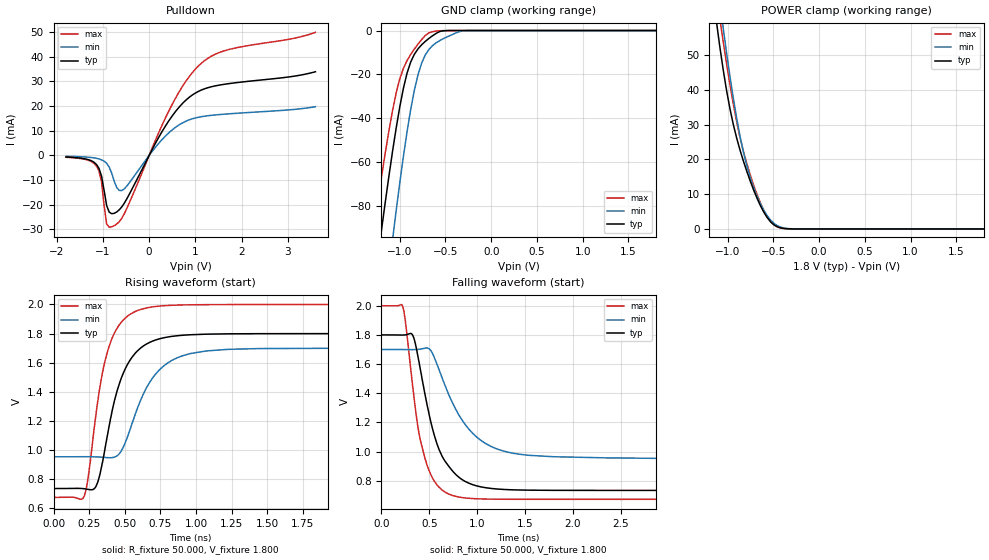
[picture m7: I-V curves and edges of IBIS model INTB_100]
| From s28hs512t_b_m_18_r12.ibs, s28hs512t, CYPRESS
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|   Model INTB_100
[Model] INTB_100
Model_type Open_drain
Polarity   Inverting
Enable   Active-High
Vmeas =  0.900V
Cref =   15.0000pF
Rref =   6.2000k
Vref =   1.8000V
C_comp   5.334pF   5.23pF   5.767pF
[Temperature Range]   25.000   0.125k   -40.000
[Voltage Range]   1.800V   1.700V   2.000V
[Pullup Reference]   1.800V   1.700V   2.000V
[Pulldown Reference]   0.0V   0.0V   0.0V
[POWER Clamp Reference]   1.800V   1.700V   2.000V
[GND Clamp Reference]   0.0V   0.0V   0.0V
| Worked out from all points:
|   slope of the pulldown table from 0 to 0.27 V, typ, clamps not added: 28.8 ohm
|   GND clamp passes 1 mA (typ) near -0.59 V on its own axis
|   POWER clamp passes 1 mA (typ) near -0.48 V on its own axis
|   rising waveform, R_fixture 50.000, V_fixture 1.800: 20-80 % time 169ps typ, 219ps min, 138ps max; typ from 0.734 V to 1.8 V
|   falling waveform, R_fixture 50.000, V_fixture 1.800: 20-80 % time 252ps typ, 383ps min, 184ps max; typ from 1.8 V to 0.734 V
[Pulldown]
|Voltage   I(typ)   I(min)   I(max)
-1.8V     -643.1uA   -344uA     -754.9uA
-1.14V    -3.675mA   -1.183mA   -4.301mA
-1.03V    -8.433mA   -1.79mA    -10.89mA
-920mV    -20.33mA   -3.208mA   -27.82mA
-755mV    -23.48mA   -10.51mA   -28.49mA
-645mV    -22.02mA   -14.2mA    -26.81mA
-535mV    -19.28mA   -13.5mA    -23.52mA
400mV     13.3mA     8.7mA      17.03mA
730mV     21.23mA    13.26mA    28.24mA
1.06V     25.89mA    15.44mA    36.14mA
1.665V    28.94mA    16.78mA    42.62mA
3.6V      33.92mA    19.74mA    49.9mA
[GND_clamp]
|Voltage   I(typ)   I(min)   I(max)
-1.8V     -294mA     -373mA     -247.3mA
-1.28V    -116.8mA   -168.5mA   -89.46mA
-1.2V     -91.34mA   -138.7mA   -67.04mA
-1.08V    -55.6mA    -96.11mA   -36.91mA
-1.04V    -44.83mA   -82.66mA   -28.74mA
-1V       -34.98mA   -69.76mA   -22.14mA
-920mV    -19.48mA   -46.23mA   -13.73mA
-800mV    -8.377mA   -20.18mA   -6.205mA
-680mV    -3.579mA   -8.59mA    -1.029mA
-560mV    -408.3uA   -4.544mA   -113.8uA
-280mV    -162.8nA   -73.51uA   -82.13nA
1.8V      272.8pA    325nA      188.3pA
[POWER_clamp]
|Voltage   I(typ)   I(min)   I(max)
-1.8V     236.7mA    239.1mA    251.1mA
-1.123V   59.68mA    73.25mA    67.66mA
-1.086V   52.46mA    65.42mA    60.6mA
-1.049V   45.83mA    57.89mA    53.9mA
-938mV    30.03mA    37.57mA    35.87mA
-864mV    22.62mA    26.6mA     26.18mA
-790mV    16.52mA    18.14mA    18.76mA
-716mV    11.21mA    11.92mA    12.63mA
-642mV    6.708mA    7.258mA    7.47mA
-494mV    1.178mA    1.619mA    1.205mA
-272mV    6.291uA    28.11uA    4.439uA
1.8V      0A         0A         0A
[Ramp]
| variable   typ   min   max
dV/dt_r   0.552/0.275n   0.438/0.373n   0.698/0.204n
dV/dt_f   0.639/0.252n   0.448/0.383n   0.796/0.184n
R_load = 50.000
[Rising Waveform]
R_fixture= 50.000
V_fixture= 1.800
V_fixture_min= 1.700
V_fixture_max= 2.000
|time   V(typ)   V(min)   V(max)
0s        734.5mV    952.8mV    673.4mV
215ps     733.3mV    953.4mV    681.2mV
296ps     745.7mV    952.2mV    1.229V
352ps     957.6mV    948.9mV    1.572V
418ps     1.297V     948.2mV    1.784V
522ps     1.593V     1.098V     1.922V
652ps     1.728V     1.427V     1.976V
873ps     1.786V     1.635V     1.996V
1.223ns   1.798V     1.691V     1.999V
6ns       1.8V       1.7V       2V
[Falling Waveform]
R_fixture= 50.000
V_fixture= 1.800
V_fixture_min= 1.700
V_fixture_max= 2.000
|time   V(typ)   V(min)   V(max)
0s        1.8V       1.7V       2V
224ps     1.799V     1.7V       1.993V
325ps     1.799V     1.699V     1.454V
391ps     1.618V     1.701V     1.13V
476ps     1.323V     1.711V     908.3mV
583ps     1.048V     1.594V     770.1mV
723ps     883.4mV    1.361V     704.3mV
993ps     765.9mV    1.101V     677.3mV
1.433ns   737.5mV    982.9mV    673.6mV
6ns       734.5mV    952.8mV    673.4mV
